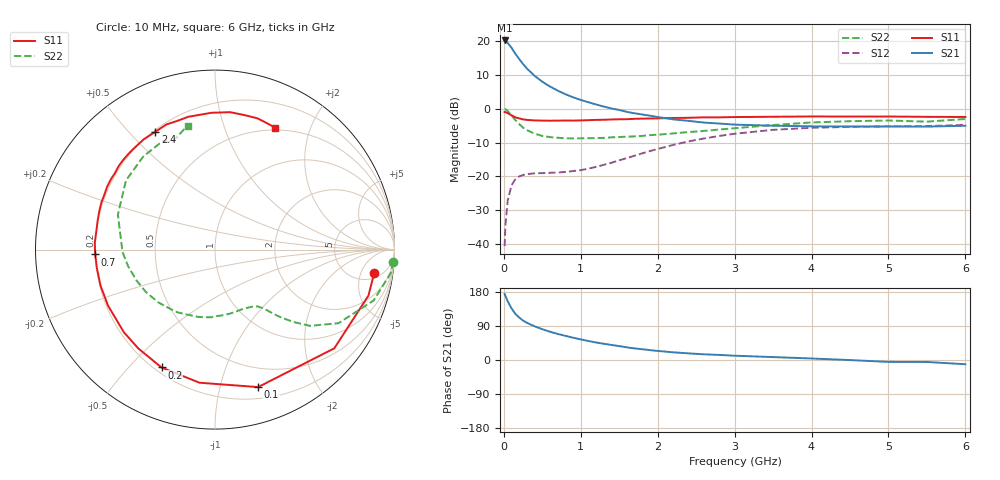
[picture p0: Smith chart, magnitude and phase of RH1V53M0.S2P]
! SIEMENS Small Signal Semiconductors
! BFR106
! Si NPN RF Bipolar Junction Transistor in SOT23
! VCE = 1.5 V  IC = 3 mA
! Common Emitter S-Parameters:  August  1996
# GHz  S  MA  R  50
!  f  S11  S21  S12  S22
! GHz  MAG  ANG  MAG  ANG  MAG  ANG  MAG  ANG
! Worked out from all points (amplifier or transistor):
!   36 points, 10 MHz to 6 GHz, reference 50 ohm
!   highest |S21| = 20.3 dB at 10 MHz (marker M1)
!   |S21| within 3 dB of that: start of sweep to 123.1 MHz
!   unconditionally stable (mu >= 1): 697.9 MHz to 2.437 GHz; 3.167 GHz to end of sweep
!   at 250 MHz: K = 0.40, MSG = 16.4 dB, |S12| = -19.6 dB
!   at 1.4 GHz: K = 1.25, MAG = 5.0 dB, |S12| = -16.0 dB
!   at 6 GHz: K = 1.02, MAG = -1.1 dB, |S12| = -4.8 dB
!   S11 on the Smith chart (normalised r, x): 10 MHz: 7, -9; 100 MHz: 0.31, -1.32; 200 MHz: 0.23, -0.62; 700 MHz: 0.20, -0.02; 2.4 GHz: 0.21, +0.60; 6 GHz: 0.47, +1.50
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0.01  0.8966 -8.4  10.31 174.2  0.0092 85.9  0.9932 -3.9
0.02  0.8925 -16.7  10.16 169.9  0.0184 80.8  0.9883 -7.6
0.05  0.8627 -39.6  9.448 155.0  0.0436 68.7  0.9279 -17.8
0.1  0.8028 -72.6  8.03 136.3  0.074 53.4  0.8009 -30.8
0.15  0.7467 -96.6  6.538 121.6  0.0904 42.4  0.6794 -38.7
0.2  0.7212 -114.4  5.468 112.0  0.0997 36.2  0.5929 -42.8
0.25  0.697 -127.8  4.607 103.9  0.1044 31.8  0.5241 -45.9
0.3  0.6855 -137.8  3.954 98.2  0.1076 29.8  0.4835 -47.7
0.4  0.6728 -152.3  3.087 88.9  0.1106 27.1  0.4272 -50.3
0.5  0.6686 -162.5  2.519 81.2  0.1115 27.0  0.3963 -53.0
0.6  0.6662 -171.2  2.141 74.6  0.1127 28.3  0.381 -56.4
0.7  0.668 -177.7  1.864 68.8  0.1136 30.6  0.3723 -60.3
0.9  0.6689 171.6  1.483 58.8  0.1194 36.7  0.364 -68.3
1.1  0.679 161.8  1.251 50.1  0.1298 43.8  0.3664 -78.2
1.6  0.7017 142.6  0.9 33.4  0.1864 55.2  0.3866 -104.2
2.2  0.7314 123.0  0.698 20.3  0.2912 53.5  0.4316 -137.0
2.4  0.7359 116.8  0.663 17.5  0.3286 50.6  0.452 -148.6
3.5  0.7625 91.5  0.562 7.7  0.4879 28.7  0.5751 160.2
4.5  0.7672 77.4  0.547 -0.2  0.5397 10.2  0.6548 127.6
5  0.7687 72.0  0.547 -5.0  0.5487 3.2  0.6709 115.8
5.5  0.7606 66.9  0.545 -5.2  0.5559 0.0  0.6451 111.9
6  0.757 63.7  0.561 -11.2  0.5777 -7.4  0.7068 102.5
